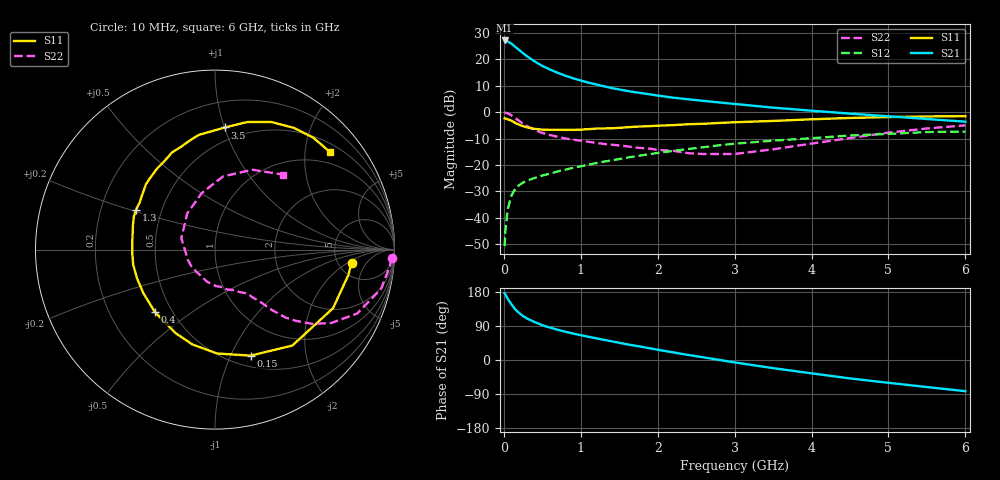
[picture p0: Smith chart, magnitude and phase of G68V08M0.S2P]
! SIEMENS Small Signal Semiconductors
! BFG193
! Si NPN RF Bipolar Junction Transistor in SOT223
! VCE = 8 V  IC = 8 mA
! Common Emitter S-Parameters:  August  1996
# GHz  S  MA  R  50
!  f  S11  S21  S12  S22
! GHz  MAG  ANG  MAG  ANG  MAG  ANG  MAG  ANG
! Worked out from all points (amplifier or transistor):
!   36 points, 10 MHz to 6 GHz, reference 50 ohm
!   highest |S21| = 27.2 dB at 10 MHz (marker M1)
!   |S21| within 3 dB of that: start of sweep to 172.1 MHz
!   unconditionally stable (mu >= 1): 976.1 MHz to 2.518 GHz
!   at 250 MHz: K = 0.46, MSG = 24.5 dB, |S12| = -26.7 dB
!   at 1.4 GHz: K = 1.07, MAG = 12.0 dB, |S12| = -18.3 dB
!   at 6 GHz: K = 0.85, MSG = 1.9 dB, |S12| = -7.3 dB
!   S11 on the Smith chart (normalised r, x): 10 MHz: 6.67, -2.31; 150 MHz: 0.62, -1.19; 400 MHz: 0.40, -0.37; 1.3 GHz: 0.36, +0.21; 3.5 GHz: 0.39, +1.00; 6 GHz: 0.69, +2.57
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0.01  0.7644 -5.4  22.82 175.8  0.0029 89.2  0.9858 -2.7
0.02  0.7567 -10.7  22.59 173.0  0.0056 85.6  0.9787 -5.4
0.05  0.7342 -26.4  21.88 161.2  0.0145 76.4  0.9514 -13.2
0.1  0.6867 -51.1  19.79 146.8  0.0266 67.7  0.8686 -24.2
0.15  0.6233 -71.4  17.12 133.2  0.0353 59.1  0.7657 -32.3
0.2  0.579 -88.8  15.01 124.0  0.0416 54.5  0.6812 -37.4
0.25  0.5433 -103.4  13.06 115.8  0.0465 50.9  0.6015 -41.3
0.3  0.5143 -115.3  11.47 109.6  0.0505 49.5  0.5466 -43.9
0.4  0.4832 -133.7  9.156 100.2  0.0568 47.2  0.4603 -46.8
0.5  0.4672 -148.8  7.519 91.8  0.063 46.8  0.4047 -48.4
0.6  0.463 -159.7  6.416 85.5  0.0687 47.0  0.3686 -49.8
0.7  0.4635 -169.6  5.571 79.7  0.0754 47.6  0.3422 -51.6
0.9  0.4625 175.4  4.388 69.8  0.0883 47.6  0.3015 -54.1
1.1  0.477 163.4  3.632 61.3  0.1013 47.3  0.275 -59.6
1.3  0.4923 153.2  3.095 53.2  0.1157 46.1  0.2504 -64.4
1.6  0.5174 139.9  2.527 41.4  0.1376 43.0  0.2255 -75.1
2.2  0.5685 119.5  1.883 20.1  0.185 34.7  0.1853 -103.5
2.8  0.6248 102.8  1.528 0.2  0.2361 23.9  0.1611 -144.3
3.5  0.6825 85.4  1.218 -21.5  0.289 8.6  0.1981 161.2
4.5  0.7771 66.2  0.939 -48.6  0.3613 -11.3  0.3234 103.2
5.5  0.8299 48.7  0.743 -71.4  0.4204 -36.2  0.4913 64.9
6  0.8405 40.2  0.66 -82.3  0.4294 -50.6  0.5635 47.9
